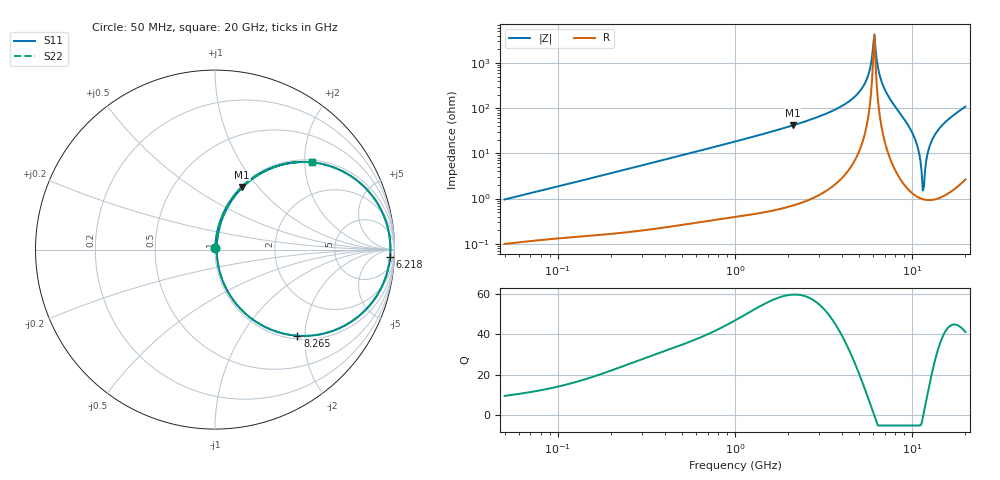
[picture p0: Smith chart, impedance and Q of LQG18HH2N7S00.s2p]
!Murata Part Number: LQG18HH2N7S00
!These Parameters are Measured in Series Mode Connection
!  o--[Z]--o
!Port1  Port2
!  o-------o
!Freq. Start=50[MHz] Stop=20[GHz], 401[Steps]
# Hz S RI R 50
!Freq.(Hz) S11(Real) S11(Imag) S21(Real) S21(Imag) S12(Real) S12(Imag) S22(Real) S22(Imag)
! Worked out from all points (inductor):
!   401 points, 50 MHz to 20 GHz, reference 50 ohm
!   read as one part in series: L = 2.99 nH near 51.52 MHz
!   highest Q = 59.5 at 2.115 GHz (marker M1), where L = 3.12 nH
!   self-resonance near 6.034 GHz
!   S11 on the Smith chart (normalised r, x): 50 MHz: 1.00, +0.02; 6.218 GHz: 21, -36; 8.265 GHz: 1.07, -1.83; 20 GHz: 1.05, +2.16
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5e7  0.00108 0.00946  0.9989 -0.00946  0.9989 -0.00946  0.00108 0.00946
1.364002e8  0.00207 0.025  0.9979 -0.025  0.9979 -0.025  0.00207 0.025
3.721004e8  0.00669 0.0668  0.9933 -0.0668  0.9933 -0.0668  0.00669 0.0668
1e9  0.0356 0.175  0.9644 -0.175  0.9644 -0.175  0.0356 0.175
2.114743e9  0.1505 0.3493  0.8495 -0.3493  0.8495 -0.3493  0.1505 0.3493
2.728004e9  0.2519 0.4255  0.7481 -0.4255  0.7481 -0.4255  0.2519 0.4255
3.908127e9  0.5245 0.4874  0.4755 -0.4874  0.4755 -0.4874  0.5245 0.4874
4.89267e9  0.7929 0.384  0.2071 -0.384  0.2071 -0.384  0.7929 0.384
5.515528e9  0.9274 0.218  0.0726 -0.218  0.0726 -0.218  0.9274 0.218
6.034176e9  0.9768 0.0309  0.0232 -0.0309  0.0232 -0.0309  0.9768 0.0309
6.217679e9  0.9756 -0.0402  0.0244 0.0402  0.0244 0.0402  0.9756 -0.0402
6.701223e9  0.9226 -0.221  0.0774 0.221  0.0774 0.221  0.9226 -0.221
7.442007e9  0.7284 -0.4203  0.2716 0.4203  0.2716 0.4203  0.7284 -0.4203
8.264682e9  0.4589 -0.48  0.5411 0.48  0.5411 0.48  0.4589 -0.48
1.034674e10  0.0545 -0.201  0.9455 0.201  0.9455 0.201  0.0545 -0.201
1.082228e10  0.0251 -0.1191  0.9749 0.1191  0.9749 0.1191  0.0251 -0.1191
1.149051e10  0.00971 -0.0112  0.9903 0.0112  0.9903 0.0112  0.00971 -0.0112
1.183995e10  0.011 0.0408  0.989 -0.0408  0.989 -0.0408  0.011 0.0408
1.257102e10  0.029 0.1388  0.971 -0.1388  0.971 -0.1388  0.029 0.1388
1.354865e10  0.0754 0.2468  0.9246 -0.2468  0.9246 -0.2468  0.0754 0.2468
1.597544e10  0.2428 0.4174  0.7572 -0.4174  0.7572 -0.4174  0.2428 0.4174
2e10  0.5387 0.4865  0.4613 -0.4865  0.4613 -0.4865  0.5387 0.4865
